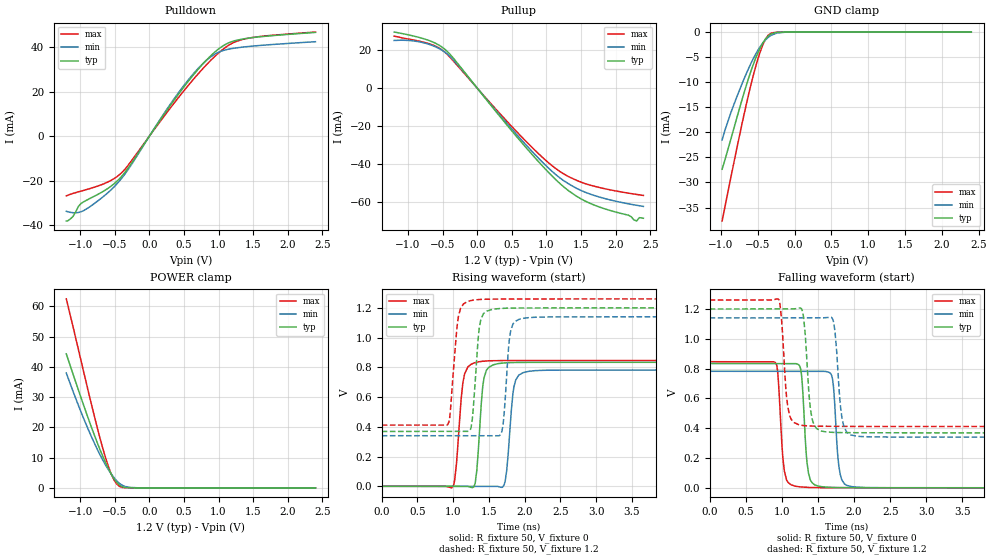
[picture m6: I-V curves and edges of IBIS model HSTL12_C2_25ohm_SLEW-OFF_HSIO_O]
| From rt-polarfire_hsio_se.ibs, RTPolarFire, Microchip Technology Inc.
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|   Model HSTL12_C2_25ohm_SLEW-OFF_HSIO_O
[Model]   HSTL12_C2_25ohm_SLEW-OFF_HSIO_O
Model_type   Output
Polarity   Non-Inverting
Enable   Active-High
Vmeas =   0.6
Cref =   5p
Rref =   50
Vref =   0.6
|   typ   min   max
C_comp_pullup   1.335e-12   1.335e-12   1.380e-12
C_comp_pulldown  1.335e-12   1.335e-12   1.380e-12
[Temperature Range]  25C   125C   -55C
[Voltage Range]  1.2   1.14   1.26
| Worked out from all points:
|   slope of the pulldown table from 0 to 0.18 V, typ, clamps not added: 21.7 ohm
|   slope of the pullup table from 0 to 0.18 V, typ, clamps not added: 21.7 ohm
|   GND clamp passes 1 mA (typ) near -0.37 V on its own axis
|   POWER clamp passes 1 mA (typ) near -0.44 V on its own axis
|   rising waveform, R_fixture 50, V_fixture 0: 20-80 % time 72.7ps typ, 78.4ps min, 82.6ps max; typ from 0 V to 0.834 V
|   rising waveform, R_fixture 50, V_fixture 1.2: 20-80 % time 75.7ps typ, 69.9ps min, 85.6ps max; typ from 0.369 V to 1.2 V
|   falling waveform, R_fixture 50, V_fixture 0: 20-80 % time 62.4ps typ, 63.3ps min, 64.1ps max; typ from 0.834 V to 0 V
|   falling waveform, R_fixture 50, V_fixture 1.2: 20-80 % time 71.8ps typ, 76ps min, 71.2ps max; typ from 1.2 V to 0.369 V
[GND Clamp]
| Voltage   I(typ)   I(min)   I(max)
-984.4mV  -27.36mA   -21.51mA   -37.68mA
-866.2mV  -21.39mA   -16.1mA    -29.03mA
-787.5mV  -17.26mA   -13.03mA   -23.38mA
-669.4mV  -11.29mA   -8.751mA   -15.31mA
-590.6mV  -7.694mA   -6.183mA   -10.37mA
-511.9mV  -4.598mA   -3.964mA   -6.023mA
-472.5mV  -3.303mA   -3.022mA   -4.164mA
-393.7mV  -1.354mA   -1.536mA   -1.373mA
-354.4mV  -738.1uA   -1.006mA   -579.2uA
-236.2mV  -56.59uA   -184.9uA   -12.91uA
-118.1mV  -2.32uA    -19uA      -220.7nA
2.4V      0A         0A         0A
[POWER Clamp]
| Voltage   I(typ)   I(min)   I(max)
-1.2V     44.33mA    38.01mA    62.52mA
-1.063V   34.96mA    29.56mA    49.5mA
-905.6mV  24.47mA    20.57mA    34.21mA
-787.5mV  17.03mA    14.47mA    23.07mA
-669.4mV  10.26mA    9.06mA     12.82mA
-590.6mV  6.299mA    5.966mA    6.995mA
-551.3mV  4.569mA    4.604mA    4.604mA
-472.5mV  1.839mA    2.331mA    1.325mA
-433.1mV  941.2uA    1.473mA    512.6uA
-354.4mV  127.4uA    466.4uA    28.07uA
-157.5mV  613.8nA    9.044uA    471.7nA
2.4V      0A         0A         0A
[Pullup]
| Voltage   I(typ)   I(min)   I(max)
-1.2V     29.74mA    25.28mA    27.57mA
-787.5mV  26.34mA    24.15mA    24.47mA
-590.6mV  23.56mA    21.7mA     22.05mA
-433.1mV  19.46mA    18.13mA    17.85mA
675mV     -30.18mA   -28.85mA   -27.05mA
1.012V    -43.93mA   -41.72mA   -38.94mA
1.239V    -51.93mA   -48.74mA   -45.18mA
1.673V    -61.62mA   -56.59mA   -51.74mA
2.184V    -67.25mA   -61.23mA   -55.58mA
2.303V    -70.33mA   -62.01mA   -56.26mA
2.342V    -68.54mA   -62.26mA   -56.47mA
2.4V      -68.87mA   -62.61mA   -56.79mA
[Pulldown]
| Voltage   I(typ)   I(min)   I(max)
-1.2V     -38.08mA   -33.71mA   -26.81mA
-1.103V   -36mA      -34.36mA   -25.69mA
-1.024V   -31.46mA   -34.24mA   -24.97mA
-945mV    -29.39mA   -33.35mA   -24.28mA
-590.6mV  -23.28mA   -25.15mA   -20.44mA
-393.7mV  -17.81mA   -18.66mA   -16.22mA
525mV     23.14mA    23.8mA     21.39mA
787.5mV   32.94mA    33.02mA    30.84mA
1.012V    39.46mA    37.87mA    37.7mA
1.2V      42.56mA    39.4mA     41.8mA
1.357V    43.7mA     40.05mA    43.56mA
2.4V      46.61mA    42.43mA    46.78mA
[Ramp]
dV/dt_r   0.500397/72.7051p  0.469176/78.3637p  0.507795/82.6387p
dV/dt_f   0.498858/71.8315p  0.479979/75.9724p  0.509267/71.2129p
R_load = 50
[Rising Waveform]
R_fixture = 50
V_fixture = 0
V_fixture_min = 0
V_fixture_max = 0
| Time   V(typ)   V(min)   V(max)
0s        1.236uV    2.004uV    1.701uV
1.002ns   -407.5uV   -445uV     2.121mV
1.159ns   -471.6uV   -515.1uV   755mV
1.289ns   -3.846mV   -573.1uV   828.3mV
1.346ns   209.1mV    -598.5uV   836.1mV
1.464ns   780.1mV    -651.2uV   842.3mV
1.712ns   829.1mV    9.695mV    845.4mV
1.849ns   832.1mV    668.6mV    845.5mV
2.054ns   832.9mV    772.6mV    845.5mV
10ns      834mV      782mV      846.3mV
[Rising Waveform]
R_fixture = 50
V_fixture = 1.2
V_fixture_min = 1.14
V_fixture_max = 1.26
| Time   V(typ)   V(min)   V(max)
0s        368.6mV    340mV      411.2mV
924ps     369.2mV    339.9mV    415.4mV
1.073ns   369.3mV    339.9mV    1.143V
1.246ns   390.1mV    339.8mV    1.248V
1.364ns   1.064V     339.8mV    1.256V
1.543ns   1.189V     339.8mV    1.258V
1.682ns   1.196V     372mV      1.259V
1.807ns   1.198V     1.053V     1.259V
1.979ns   1.199V     1.129V     1.259V
10ns      1.2V       1.14V      1.26V
[Falling Waveform]
R_fixture = 50
V_fixture = 0
V_fixture_min = 0
V_fixture_max = 0
| Time   V(typ)   V(min)   V(max)
0s        834mV      782mV      846.3mV
916ps     833.4mV    781.8mV    836mV
1.035ns   833.3mV    781.7mV    111.3mV
1.188ns   833.2mV    781.7mV    11.05mV
1.368ns   99.98mV    781.7mV    2.994mV
1.507ns   11.4mV     781.6mV    1.668mV
1.69ns    3.287mV    752.7mV    1.235mV
1.807ns   1.712mV    92.26mV    1.039mV
1.968ns   1.125mV    8.229mV    769.3uV
10ns      2.047uV    2.888uV    2.148uV
[Falling Waveform]
R_fixture = 50
V_fixture = 1.2
V_fixture_min = 1.14
V_fixture_max = 1.26
| Time   V(typ)   V(min)   V(max)
0s        1.2V       1.14V      1.26V
952ps     1.201V     1.141V     1.266V
1.082ns   1.201V     1.141V     543.1mV
1.239ns   1.206V     1.141V     422.5mV
1.418ns   464.1mV    1.141V     414.6mV
1.543ns   381.6mV    1.141V     413.3mV
1.707ns   372.3mV    1.128V     412.8mV
1.833ns   370.7mV    466.6mV    412.5mV
2.041ns   369.9mV    346.3mV    412.1mV
10ns      368.6mV    340mV      411.2mV
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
